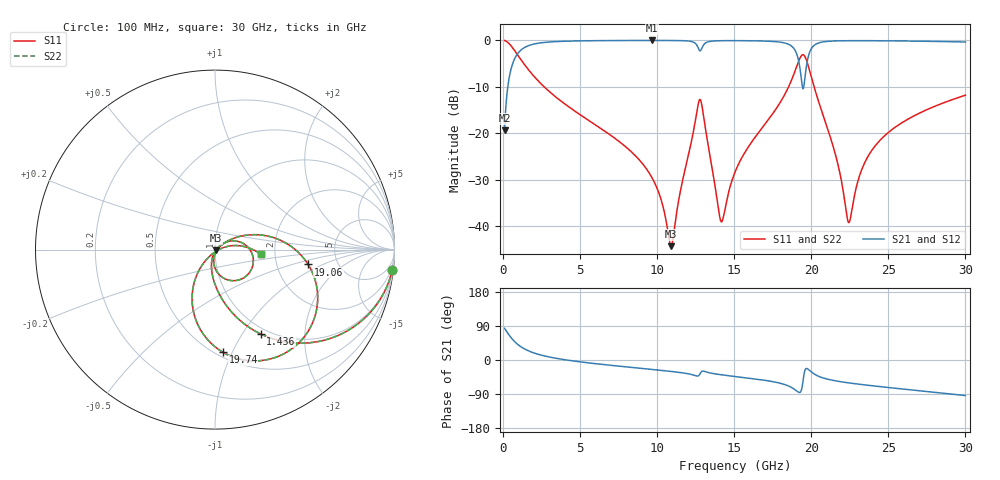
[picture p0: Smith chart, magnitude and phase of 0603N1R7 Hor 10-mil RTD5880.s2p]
# GHz S MA R 50
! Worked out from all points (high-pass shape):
!   3201 points, 100 MHz to 30 GHz, reference 50 ohm
!   highest |S21| = -0.04 dB at 9.687 GHz (marker M1); lowest = -19.3 dB at 100 MHz (marker M2)
!   |S21| within 3 dB of the highest: 910.1 MHz to 19.07 GHz (18.16 GHz wide, 182 % of centre); 19.84 GHz to end of sweep
!   lowest |S11| = -44.3 dB at 10.9 GHz (marker M3), VSWR 1.01, Z = 50.5 - j0.359 ohm
!   |S11| at or under -10 dB: 2.663 GHz to 18.53 GHz (15.87 GHz wide, 150 % of centre); 20.18 GHz to end of sweep
!   |S22| runs from -44.3 to -0.1 dB; largest |S21 - S12| = 0
!   S11 on the Smith chart (normalised r, x): 100 MHz: 1, -18; 1.436 GHz: 0.92, -1.21; 19.06 GHz: 3.04, -0.69; 19.74 GHz: 0.54, -0.92; 30 GHz: 1.68, -0.09
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0.1  0.9941 -6.5  0.1082 83.5  0.1082 83.5  0.9941 -6.5
0.5671875  0.8504 -33.3  0.5254 56.7  0.5254 56.7  0.8504 -33.3
1.436156  0.535 -61.5  0.8435 28.3  0.8435 28.3  0.535 -61.5
5.089563  0.1548 -94.3  0.9852 -5.3  0.9852 -5.3  0.1548 -94.3
9.686687  0.03278 -107.2  0.9949 -25.0  0.9949 -25.0  0.03278 -107.2
10.06978  0.02382 -105.0  0.9948 -26.6  0.9948 -26.6  0.02382 -105.0
10.90137  0.006124 -35.5  0.9937 -30.2  0.9937 -30.2  0.006124 -35.5
12.40572  0.117 24.6  0.9447 -40.3  0.9447 -40.3  0.117 24.6
12.74209  0.2284 -22.8  0.7782 -38.8  0.7782 -38.8  0.2284 -22.8
13.17191  0.1019 -90.2  0.9434 -31.3  0.9434 -31.3  0.1019 -90.2
14.12497  0.01143 -43.8  0.9884 -38.8  0.9884 -38.8  0.01143 -43.8
15.05  0.03824 33.1  0.9902 -43.4  0.9902 -43.4  0.03824 33.1
17.82509  0.1952 24.4  0.961 -59.8  0.961 -59.8  0.1952 24.4
19.05847  0.5254 -9.1  0.7098 -81.9  0.7098 -81.9  0.5254 -9.1
19.45091  0.6995 -50.0  0.303 -59.3  0.303 -59.3  0.6995 -50.0
19.74056  0.5735 -85.6  0.5972 -22.9  0.5972 -22.9  0.5735 -85.6
20.03956  0.3831 -107.5  0.8288 -32.6  0.8288 -32.6  0.3831 -107.5
21.59997  0.05639 -130.0  0.9835 -55.2  0.9835 -55.2  0.05639 -130.0
22.42222  0.01099 -61.3  0.9887 -60.4  0.9887 -60.4  0.01099 -61.3
23.44069  0.0473 13.1  0.9893 -65.6  0.9893 -65.6  0.0473 13.1
25.01978  0.1026 12.5  0.9859 -72.7  0.9859 -72.7  0.1026 12.5
30  0.2567 -5.8  0.9571 -93.8  0.9571 -93.8  0.2567 -5.8
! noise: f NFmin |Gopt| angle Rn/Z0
0.1  0.0006067  0.9612  0.7067  0.003532
3.417  0.004047  0.8105  9.88  0.004419
6.743  0.006857  0.7835  18.97  0.00633
10.06  0.01022  0.7847  27.94  0.009196
13.39  0.02877  0.8931  36.9  0.05279
16.7  0.01982  0.8163  45.54  0.01921
20.03  0.07165  0.9359  54.34  0.1971
23.35  0.02139  0.7735  62.6  0.01417
26.67  0.02175  0.7519  70.53  0.01191
30  0.02399  0.7505  78.27  0.01181
